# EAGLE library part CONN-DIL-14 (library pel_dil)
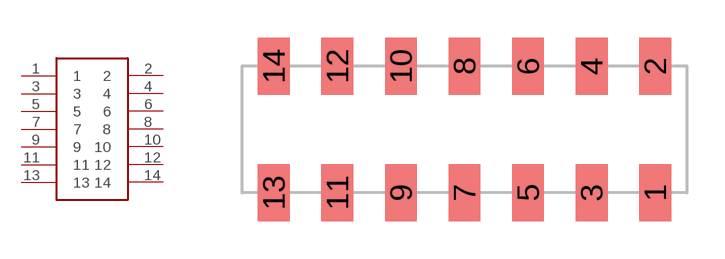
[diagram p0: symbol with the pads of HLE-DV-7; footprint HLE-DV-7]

Designator prefix X

## CONN-DIL-14-HLE-DV  [HLE-DV-7]
1  1
2  2
3  3
4  4
5  5
6  6
7  7
8  8
9  9
10  10
11  11
12  12
13  13
14  14

## Footprint HLE-DV-7 (pad centres in mm)
smd 1.27 x 2.29: 1 7.62,-2.527; 2 7.62,2.527; 3 5.08,-2.527; 4 5.08,2.527; 5 2.54,-2.527; 6 2.54,2.527; 7 0,-2.527; 8 0,2.527; 9 -2.54,-2.527; 10 -2.54,2.527; 11 -5.08,-2.527; 12 -5.08,2.527; 13 -7.62,-2.527; 14 -7.62,2.527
